| IBIS File LibisMaker.ibs
| LibisGen v2.0.1.0, 02/25/2008, Lattice Semiconductor Corporation
| Modified by LibisMaker v2.0.1.0, 02/25/2008, Lattice Semiconductor
| North Carolina State University, ERL, 2006
[IBIS ver]   3.2
[File name]   lptm21.ibs
[File Rev]   1.0
[Date]   May 27, 2015
[Source]   Lattice Semiconductor cs200fl Process
[Notes]   Device: LPTM21   Final
   Lattice Semiconductor has worked hard to ensure the
   models below are accurate and complete.  However, the
   data below was generated using simulation of the
   input/output model files for the silicon.  Therefore,
   the data below is for reference and initial design
   purposes only.
   Lattice Semiconductor grants permission to use this
   data for use in printed circuit design using this
   Lattice programmable logic device.  Other use of this
   code, including the selling or duplication of any
   portion is strictly prohibited.
|   NAMING CONVENTION
   The IBIS [Model] header is limited by the specification to a
   total of characters.  With such a set of characters available
   for naming models it becomes important to attempt to
   meaningfully encode the IO standards so they fit within the
   twenty character limit.  It would seem that twenty characters
   would provide room enough for describing IO's.  However, the
   PLD IO structure continues to grow more and more complex.  The
   complexity is making the twenty characters insuffiently
   descriptive.  In order to overcome this issue the naming
   convention described below is implemented to resolve the issue.
The twenty character space is managed as follows:
   bbbvvvsdddprugtcoixx
   b = standard
   v = voltage (x.xx V)
   s = slew code
   d = drive (xx.x ma)
   p = pullup code
   r = series resistance  or bank_vccio code
   u = terminate to vcc code
   g = terminate to gnd code
   t = terminate to vtt code
   c = common mode termination mode
   o = diff resistor code
   i = diff resistor current code
   x = reserved
   standard
   lvcmos   lvc
   lvcmosd   lvd
   lvcmosr   lvr
   lvds25e   lve
   lvttl   lvt
   lvttld   ltd
   pci   pci
   sstl_I   ss1
   sstl_II   ss2
   sstld_I   s1d
   sstld_II   s2d
   hstl_i   hs1
   hstl_ii   hs2
   hstld_i   h1d
   hstld_ii   h2d
   lvds25   lvs
   blvds25   blv
   blvds25e   blv
   mlvds25   mlv
   mlvds25e   mlv
   lvpecl33   lvp
   lvpecl33e   lvp
   rsds25   rsd
   rsds25e   rse
   mipi   mip
   mipi_lp   mip
   vref1   vr1
   vref2   vr2
   ref_res   rer
   slew
   na   a
   fast   f
   slow   s
   pullmode
   off   a
   pullup   b
   pulldown   c
   bushold   d
   clamp   e
   up_clamp   f
   down_clamp   g
   keeper_clamp   h
   impedance or Bank_vccio
   off   a
   25   b
   33   c
   50   d
   100   e
   3.3   f
   2.5   g
   1.8   h
   1.5   i
   1.2   j
   termVCC
   off   a
   50   b
   100   c
   120   d
   termGND
   off   a
   50   b
   100   c
   120   d
   termVTT
   off   a
   60   b
   75   c
   120   d
   150   e
   210   f
   VCMT
   off   a
   VCMT   b
   VTT   c
   DDR-2   d
   differential resistor
   off   a
   100   b
   diff drive
   NA   a
   2.0   b
   3.5   c
   1.25   f
   2.5   g
   Reserved   IO type
   in   input only
   ou   output
   io   I/O
   od   Open drain
   on   Inverting differential I/O
   (signal name only)
   op   Non-Inverting differential I/O
   (signal name only)
   Lattice Semiconductor Corporation
   5555 NE Moore Court
   Hillsboro, OR 97214
   U.S.A
   TEL: 1-800-Lattice (USA and Canada)
   408-826-6000 (other locations)
   web: http://www.latticesemi.com/
   email: techsupport@latticesemi.com
[Disclaimer] This IBIS source code is intended as a design reference
   which illustrates how the Lattice Semiconductor device operates.
   It is the user's responsibility to verify their design for
   consistency and functionality through the use of formal
   verification methods.  Lattice Semiconductor provides no warranty
   regarding the use or functionality of this data.
[Copyright]   Copyright 2007 by Lattice Semiconductor Corporation
|   Component LPTM21
[Component]   LPTM21
[Manufacturer]   Lattice Semiconductor Corp.
[Package]
|ftBGA237
| variable   typ   min   max
R_pkg   278.36m   251.54m   305.19m
L_pkg   6.04nH   3.27nH   8.79nH
C_pkg   0.509pF   0.44pF   0.704pF
[Pin] signal_name   model_name   R_pin   L_pin   C_pin
1   blv250axxxafaaaaaain   blv250axxxafaaaaaain
2   blv250axxxafaaaabain   blv250axxxafaaaabain
3   blv250axxxagaaaaaain   blv250axxxagaaaaaain
4   blv250axxxagaaaabain   blv250axxxagaaaabain
5   blv250axxxefaaaaaain   blv250axxxefaaaaaain
6   blv250axxxefaaaabain   blv250axxxefaaaabain
7   blv250axxxegaaaaaain   blv250axxxegaaaaaain
8   blv250axxxegaaaabain   blv250axxxegaaaabain
9   blv250f160aaaaaaaaio   blv250f160aaaaaaaaio
10   blv250f160aaaaaaaaop   blv250f160aaaaaaaaou
11   blv250f160aaaaaaaaon   blv250f160aaaaaaaaou
12   blv250f160eaaaaaaaio   blv250f160eaaaaaaaio
13   blv250f160eaaaaaaaop   blv250f160eaaaaaaaou
14   blv250f160eaaaaaaaon   blv250f160eaaaaaaaou
15   blv250s160aaaaaaaaio   blv250s160aaaaaaaaio
16   blv250s160aaaaaaaaop   blv250s160aaaaaaaaou
17   blv250s160aaaaaaaaon   blv250s160aaaaaaaaou
18   blv250s160eaaaaaaaio   blv250s160eaaaaaaaio
19   blv250s160eaaaaaaaop   blv250s160eaaaaaaaou
20   blv250s160eaaaaaaaon   blv250s160eaaaaaaaou
21   h1d180axxxafaaaaaain   h1d180axxxafaaaaaain
22   h1d180axxxafaaaabain   h1d180axxxafaaaabain
23   h1d180axxxagaaaaaain   h1d180axxxagaaaaaain
24   h1d180axxxagaaaabain   h1d180axxxagaaaabain
25   h1d180axxxahaaaaaain   h1d180axxxahaaaaaain
26   h1d180axxxahaaaabain   h1d180axxxahaaaabain
27   h1d180axxxefaaaaaain   h1d180axxxefaaaaaain
28   h1d180axxxefaaaabain   h1d180axxxefaaaabain
29   h1d180axxxegaaaaaain   h1d180axxxegaaaaaain
30   h1d180axxxegaaaabain   h1d180axxxegaaaabain
31   h1d180axxxehaaaaaain   h1d180axxxehaaaaaain
32   h1d180axxxehaaaabain   h1d180axxxehaaaabain
33   h1d180f080aaaaaaaaio   h1d180f080aaaaaaaaio
34   h1d180f080aaaaaaaaop   h1d180f080aaaaaaaaou
35   h1d180f080aaaaaaaaon   h1d180f080aaaaaaaaou
36   h1d180f080aaaaaabaio   h1d180f080aaaaaabaio
37   h1d180f080eaaaaaaaio   h1d180f080eaaaaaaaio
38   h1d180f080eaaaaaaaop   h1d180f080eaaaaaaaou
39   h1d180f080eaaaaaaaon   h1d180f080eaaaaaaaou
40   h1d180f080eaaaaabaio   h1d180f080eaaaaabaio
41   h1d180s080aaaaaaaaio   h1d180s080aaaaaaaaio
42   h1d180s080aaaaaaaaop   h1d180s080aaaaaaaaou
43   h1d180s080aaaaaaaaon   h1d180s080aaaaaaaaou
44   h1d180s080aaaaaabaio   h1d180s080aaaaaabaio
45   h1d180s080eaaaaaaaio   h1d180s080eaaaaaaaio
46   h1d180s080eaaaaaaaop   h1d180s080eaaaaaaaou
47   h1d180s080eaaaaaaaon   h1d180s080eaaaaaaaou
48   h1d180s080eaaaaabaio   h1d180s080eaaaaabaio
49   h2d180axxxafaaaaaain   h2d180axxxafaaaaaain
50   h2d180axxxafaaaabain   h2d180axxxafaaaabain
51   h2d180axxxagaaaaaain   h2d180axxxagaaaaaain
52   h2d180axxxagaaaabain   h2d180axxxagaaaabain
53   h2d180axxxahaaaaaain   h2d180axxxahaaaaaain
54   h2d180axxxahaaaabain   h2d180axxxahaaaabain
55   h2d180axxxefaaaaaain   h2d180axxxefaaaaaain
56   h2d180axxxefaaaabain   h2d180axxxefaaaabain
57   h2d180axxxegaaaaaain   h2d180axxxegaaaaaain
58   h2d180axxxegaaaabain   h2d180axxxegaaaabain
59   h2d180axxxehaaaaaain   h2d180axxxehaaaaaain
60   h2d180axxxehaaaabain   h2d180axxxehaaaabain
61   hs1180axxxafaaaaaain   hs1180axxxafaaaaaain
62   hs1180axxxagaaaaaain   hs1180axxxagaaaaaain
63   hs1180axxxahaaaaaain   hs1180axxxahaaaaaain
64   hs1180axxxefaaaaaain   hs1180axxxefaaaaaain
65   hs1180axxxegaaaaaain   hs1180axxxegaaaaaain
66   hs1180axxxehaaaaaain   hs1180axxxehaaaaaain
67   hs1180f080aaaaaaaaio   hs1180f080aaaaaaaaio
68   hs1180f080aaaaaaaaou   hs1180f080aaaaaaaaou
69   hs1180f080eaaaaaaaio   hs1180f080eaaaaaaaio
70   hs1180f080eaaaaaaaou   hs1180f080eaaaaaaaou
71   hs1180s080aaaaaaaaio   hs1180s080aaaaaaaaio
72   hs1180s080aaaaaaaaou   hs1180s080aaaaaaaaou
73   hs1180s080eaaaaaaaio   hs1180s080eaaaaaaaio
74   hs1180s080eaaaaaaaou   hs1180s080eaaaaaaaou
75   hs2180axxxafaaaaaain   hs2180axxxafaaaaaain
76   hs2180axxxagaaaaaain   hs2180axxxagaaaaaain
77   hs2180axxxahaaaaaain   hs2180axxxahaaaaaain
78   hs2180axxxefaaaaaain   hs2180axxxefaaaaaain
79   hs2180axxxegaaaaaain   hs2180axxxegaaaaaain
80   hs2180axxxehaaaaaain   hs2180axxxehaaaaaain
81   ltd330axxxafaaaaaain   ltd330axxxafaaaaaain
82   ltd330axxxefaaaaaain   ltd330axxxefaaaaaain
83   ltd330f040aaaaaaaaio   ltd330f040aaaaaaaaio
84   ltd330f040aaaaaaaaop   ltd330f040aaaaaaaaou
85   ltd330f040aaaaaaaaon   ltd330f040aaaaaaaaou
86   ltd330f040eaaaaaaaio   ltd330f040eaaaaaaaio
87   ltd330f040eaaaaaaaop   ltd330f040eaaaaaaaou
88   ltd330f040eaaaaaaaon   ltd330f040eaaaaaaaou
89   ltd330f080aaaaaaaaio   ltd330f080aaaaaaaaio
90   ltd330f080aaaaaaaaop   ltd330f080aaaaaaaaou
91   ltd330f080aaaaaaaaon   ltd330f080aaaaaaaaou
92   ltd330f080eaaaaaaaio   ltd330f080eaaaaaaaio
93   ltd330f080eaaaaaaaop   ltd330f080eaaaaaaaou
94   ltd330f080eaaaaaaaon   ltd330f080eaaaaaaaou
95   ltd330f120aaaaaaaaio   ltd330f120aaaaaaaaio
96   ltd330f120aaaaaaaaop   ltd330f120aaaaaaaaou
97   ltd330f120aaaaaaaaon   ltd330f120aaaaaaaaou
98   ltd330f120eaaaaaaaio   ltd330f120eaaaaaaaio
99   ltd330f120eaaaaaaaop   ltd330f120eaaaaaaaou
100  ltd330f120eaaaaaaaon   ltd330f120eaaaaaaaou
101  ltd330f160aaaaaaaaio   ltd330f160aaaaaaaaio
102  ltd330f160aaaaaaaaop   ltd330f160aaaaaaaaou
103  ltd330f160aaaaaaaaon   ltd330f160aaaaaaaaou
104  ltd330f160eaaaaaaaio   ltd330f160eaaaaaaaio
105  ltd330f160eaaaaaaaop   ltd330f160eaaaaaaaou
106  ltd330f160eaaaaaaaon   ltd330f160eaaaaaaaou
107  ltd330f240aaaaaaaaio   ltd330f240aaaaaaaaio
108  ltd330f240aaaaaaaaop   ltd330f240aaaaaaaaou
109  ltd330f240aaaaaaaaon   ltd330f240aaaaaaaaou
110  ltd330f240eaaaaaaaio   ltd330f240eaaaaaaaio
111  ltd330f240eaaaaaaaop   ltd330f240eaaaaaaaou
112  ltd330f240eaaaaaaaon   ltd330f240eaaaaaaaou
113  ltd330s040aaaaaaaaio   ltd330s040aaaaaaaaio
114  ltd330s040aaaaaaaaop   ltd330s040aaaaaaaaou
115  ltd330s040aaaaaaaaon   ltd330s040aaaaaaaaou
116  ltd330s040eaaaaaaaio   ltd330s040eaaaaaaaio
117  ltd330s040eaaaaaaaop   ltd330s040eaaaaaaaou
118  ltd330s040eaaaaaaaon   ltd330s040eaaaaaaaou
119  ltd330s080aaaaaaaaio   ltd330s080aaaaaaaaio
120  ltd330s080aaaaaaaaop   ltd330s080aaaaaaaaou
121  ltd330s080aaaaaaaaon   ltd330s080aaaaaaaaou
122  ltd330s080eaaaaaaaio   ltd330s080eaaaaaaaio
123  ltd330s080eaaaaaaaop   ltd330s080eaaaaaaaou
124  ltd330s080eaaaaaaaon   ltd330s080eaaaaaaaou
125  ltd330s120aaaaaaaaio   ltd330s120aaaaaaaaio
126  ltd330s120aaaaaaaaop   ltd330s120aaaaaaaaou
127  ltd330s120aaaaaaaaon   ltd330s120aaaaaaaaou
128  ltd330s120eaaaaaaaio   ltd330s120eaaaaaaaio
129  ltd330s120eaaaaaaaop   ltd330s120eaaaaaaaou
130  ltd330s120eaaaaaaaon   ltd330s120eaaaaaaaou
131  ltd330s160aaaaaaaaio   ltd330s160aaaaaaaaio
132  ltd330s160aaaaaaaaop   ltd330s160aaaaaaaaou
133  ltd330s160aaaaaaaaon   ltd330s160aaaaaaaaou
134  ltd330s160eaaaaaaaio   ltd330s160eaaaaaaaio
135  ltd330s160eaaaaaaaop   ltd330s160eaaaaaaaou
136  ltd330s160eaaaaaaaon   ltd330s160eaaaaaaaou
137  ltd330s240aaaaaaaaio   ltd330s240aaaaaaaaio
138  ltd330s240aaaaaaaaop   ltd330s240aaaaaaaaou
139  ltd330s240aaaaaaaaon   ltd330s240aaaaaaaaou
140  ltd330s240eaaaaaaaio   ltd330s240eaaaaaaaio
141  ltd330s240eaaaaaaaop   ltd330s240eaaaaaaaou
142  ltd330s240eaaaaaaaon   ltd330s240eaaaaaaaou
143  lvc120axxxafaaaaaain   lvc120axxxafaaaaaain
144  lvc120axxxagaaaaaain   lvc120axxxagaaaaaain
145  lvc120axxxahaaaaaain   lvc120axxxahaaaaaain
146  lvc120axxxaiaaaaaain   lvc120axxxaiaaaaaain
147  lvc120axxxbjaaaaaain   lvc120axxxbjaaaaaain
148  lvc120axxxcfaaaaaain   lvc120axxxcfaaaaaain
149  lvc120axxxcgaaaaaain   lvc120axxxcgaaaaaain
150  lvc120axxxchaaaaaain   lvc120axxxchaaaaaain
151  lvc120axxxciaaaaaain   lvc120axxxciaaaaaain
152  lvc120axxxdjaaaaaain   lvc120axxxdjaaaaaain
153  lvc120axxxefaaaaaain   lvc120axxxefaaaaaain
154  lvc120axxxegaaaaaain   lvc120axxxegaaaaaain
155  lvc120axxxehaaaaaain   lvc120axxxehaaaaaain
156  lvc120axxxeiaaaaaain   lvc120axxxeiaaaaaain
157  lvc120axxxejaaaaaain   lvc120axxxejaaaaaain
158  lvc120axxxfjaaaaaain   lvc120axxxfjaaaaaain
159  lvc120axxxgfaaaaaain   lvc120axxxgfaaaaaain
160  lvc120axxxggaaaaaain   lvc120axxxggaaaaaain
161  lvc120axxxghaaaaaain   lvc120axxxghaaaaaain
162  lvc120axxxgiaaaaaain   lvc120axxxgiaaaaaain
163  lvc120axxxgjaaaaaain   lvc120axxxgjaaaaaain
164  lvc120axxxhjaaaaaain   lvc120axxxhjaaaaaain
165  lvc120f020aaaaaaaaio   lvc120f020aaaaaaaaio
166  lvc120f020aaaaaaaaou   lvc120f020aaaaaaaaou
167  lvc120f020baaaaaaaio   lvc120f020baaaaaaaio
168  lvc120f020baaaaaaaou   lvc120f020baaaaaaaou
169  lvc120f020caaaaaaaio   lvc120f020caaaaaaaio
170  lvc120f020caaaaaaaou   lvc120f020caaaaaaaou
171  lvc120f020daaaaaaaio   lvc120f020daaaaaaaio
172  lvc120f020daaaaaaaou   lvc120f020daaaaaaaou
173  lvc120f020eaaaaaaaio   lvc120f020eaaaaaaaio
174  lvc120f020eaaaaaaaou   lvc120f020eaaaaaaaou
175  lvc120f020faaaaaaaio   lvc120f020faaaaaaaio
176  lvc120f020faaaaaaaou   lvc120f020faaaaaaaou
177  lvc120f020gaaaaaaaio   lvc120f020gaaaaaaaio
178  lvc120f020gaaaaaaaou   lvc120f020gaaaaaaaou
179  lvc120f020haaaaaaaio   lvc120f020haaaaaaaio
180  lvc120f020haaaaaaaou   lvc120f020haaaaaaaou
181  lvc120f040afaaaaaaod   lvc120f040afaaaaaaod
182  lvc120f040agaaaaaaod   lvc120f040agaaaaaaod
183  lvc120f040ahaaaaaaod   lvc120f040ahaaaaaaod
184  lvc120f040aiaaaaaaod   lvc120f040aiaaaaaaod
185  lvc120f040ajaaaaaaod   lvc120f040ajaaaaaaod
186  lvc120f060aaaaaaaaio   lvc120f060aaaaaaaaio
187  lvc120f060aaaaaaaaou   lvc120f060aaaaaaaaou
188  lvc120f060baaaaaaaio   lvc120f060baaaaaaaio
189  lvc120f060baaaaaaaou   lvc120f060baaaaaaaou
190  lvc120f060caaaaaaaio   lvc120f060caaaaaaaio
191  lvc120f060caaaaaaaou   lvc120f060caaaaaaaou
192  lvc120f060daaaaaaaio   lvc120f060daaaaaaaio
193  lvc120f060daaaaaaaou   lvc120f060daaaaaaaou
194  lvc120f060eaaaaaaaio   lvc120f060eaaaaaaaio
195  lvc120f060eaaaaaaaou   lvc120f060eaaaaaaaou
196  lvc120f060faaaaaaaio   lvc120f060faaaaaaaio
197  lvc120f060faaaaaaaou   lvc120f060faaaaaaaou
198  lvc120f060gaaaaaaaio   lvc120f060gaaaaaaaio
199  lvc120f060gaaaaaaaou   lvc120f060gaaaaaaaou
200  lvc120f060haaaaaaaio   lvc120f060haaaaaaaio
201  lvc120f060haaaaaaaou   lvc120f060haaaaaaaou
202  lvc120f080afaaaaaaod   lvc120f080afaaaaaaod
203  lvc120f080agaaaaaaod   lvc120f080agaaaaaaod
204  lvc120f080ahaaaaaaod   lvc120f080ahaaaaaaod
205  lvc120f080aiaaaaaaod   lvc120f080aiaaaaaaod
206  lvc120f080ajaaaaaaod   lvc120f080ajaaaaaaod
207  lvc120f120afaaaaaaod   lvc120f120afaaaaaaod
208  lvc120f120agaaaaaaod   lvc120f120agaaaaaaod
209  lvc120f120ahaaaaaaod   lvc120f120ahaaaaaaod
210  lvc120f160afaaaaaaod   lvc120f160afaaaaaaod
211  lvc120f160agaaaaaaod   lvc120f160agaaaaaaod
212  lvc120f240afaaaaaaod   lvc120f240afaaaaaaod
213  lvc120s020aaaaaaaaio   lvc120s020aaaaaaaaio
214  lvc120s020aaaaaaaaou   lvc120s020aaaaaaaaou
215  lvc120s020baaaaaaaio   lvc120s020baaaaaaaio
216  lvc120s020baaaaaaaou   lvc120s020baaaaaaaou
217  lvc120s020caaaaaaaio   lvc120s020caaaaaaaio
218  lvc120s020caaaaaaaou   lvc120s020caaaaaaaou
219  lvc120s020daaaaaaaio   lvc120s020daaaaaaaio
220  lvc120s020daaaaaaaou   lvc120s020daaaaaaaou
221  lvc120s020eaaaaaaaio   lvc120s020eaaaaaaaio
222  lvc120s020eaaaaaaaou   lvc120s020eaaaaaaaou
223  lvc120s020faaaaaaaio   lvc120s020faaaaaaaio
224  lvc120s020faaaaaaaou   lvc120s020faaaaaaaou
225  lvc120s020gaaaaaaaio   lvc120s020gaaaaaaaio
226  lvc120s020gaaaaaaaou   lvc120s020gaaaaaaaou
227  lvc120s020haaaaaaaio   lvc120s020haaaaaaaio
228  lvc120s020haaaaaaaou   lvc120s020haaaaaaaou
229  lvc120s040afaaaaaaod   lvc120s040afaaaaaaod
230  lvc120s040agaaaaaaod   lvc120s040agaaaaaaod
231  lvc120s040ahaaaaaaod   lvc120s040ahaaaaaaod
232  lvc120s040aiaaaaaaod   lvc120s040aiaaaaaaod
233  lvc120s040ajaaaaaaod   lvc120s040ajaaaaaaod
234  lvc120s060aaaaaaaaio   lvc120s060aaaaaaaaio
235  lvc120s060aaaaaaaaou   lvc120s060aaaaaaaaou
236  lvc120s060baaaaaaaio   lvc120s060baaaaaaaio
237  lvc120s060baaaaaaaou   lvc120s060baaaaaaaou
238  lvc120s060caaaaaaaio   lvc120s060caaaaaaaio
239  lvc120s060caaaaaaaou   lvc120s060caaaaaaaou
240  lvc120s060daaaaaaaio   lvc120s060daaaaaaaio
241  lvc120s060daaaaaaaou   lvc120s060daaaaaaaou
242  lvc120s060eaaaaaaaio   lvc120s060eaaaaaaaio
243  lvc120s060eaaaaaaaou   lvc120s060eaaaaaaaou
244  lvc120s060faaaaaaaio   lvc120s060faaaaaaaio
245  lvc120s060faaaaaaaou   lvc120s060faaaaaaaou
246  lvc120s060gaaaaaaaio   lvc120s060gaaaaaaaio
247  lvc120s060gaaaaaaaou   lvc120s060gaaaaaaaou
248  lvc120s060haaaaaaaio   lvc120s060haaaaaaaio
249  lvc120s060haaaaaaaou   lvc120s060haaaaaaaou
250  lvc120s080afaaaaaaod   lvc120s080afaaaaaaod
251  lvc120s080agaaaaaaod   lvc120s080agaaaaaaod
252  lvc120s080ahaaaaaaod   lvc120s080ahaaaaaaod
253  lvc120s080aiaaaaaaod   lvc120s080aiaaaaaaod
254  lvc120s080ajaaaaaaod   lvc120s080ajaaaaaaod
255  lvc120s120afaaaaaaod   lvc120s120afaaaaaaod
256  lvc120s120agaaaaaaod   lvc120s120agaaaaaaod
257  lvc120s120ahaaaaaaod   lvc120s120ahaaaaaaod
258  lvc120s160afaaaaaaod   lvc120s160afaaaaaaod
259  lvc120s160agaaaaaaod   lvc120s160agaaaaaaod
260  lvc120s240afaaaaaaod   lvc120s240afaaaaaaod
261  lvc150axxxafaaaaaain   lvc150axxxafaaaaaain
262  lvc150axxxagaaaaaain   lvc150axxxagaaaaaain
263  lvc150axxxahaaaaaain   lvc150axxxahaaaaaain
264  lvc150axxxaiaaaaaain   lvc150axxxaiaaaaaain
265  lvc150axxxajaaaaaain   lvc150axxxajaaaaaain
266  lvc150axxxbiaaaaaain   lvc150axxxbiaaaaaain
267  lvc150axxxcfaaaaaain   lvc150axxxcfaaaaaain
268  lvc150axxxcgaaaaaain   lvc150axxxcgaaaaaain
269  lvc150axxxchaaaaaain   lvc150axxxchaaaaaain
270  lvc150axxxciaaaaaain   lvc150axxxciaaaaaain
271  lvc150axxxcjaaaaaain   lvc150axxxcjaaaaaain
272  lvc150axxxdiaaaaaain   lvc150axxxdiaaaaaain
273  lvc150axxxefaaaaaain   lvc150axxxefaaaaaain
274  lvc150axxxegaaaaaain   lvc150axxxegaaaaaain
275  lvc150axxxehaaaaaain   lvc150axxxehaaaaaain
276  lvc150axxxeiaaaaaain   lvc150axxxeiaaaaaain
277  lvc150axxxfiaaaaaain   lvc150axxxfiaaaaaain
278  lvc150axxxgfaaaaaain   lvc150axxxgfaaaaaain
279  lvc150axxxggaaaaaain   lvc150axxxggaaaaaain
280  lvc150axxxghaaaaaain   lvc150axxxghaaaaaain
281  lvc150axxxgiaaaaaain   lvc150axxxgiaaaaaain
282  lvc150axxxhiaaaaaain   lvc150axxxhiaaaaaain
283  lvc150f040aaaaaaaaio   lvc150f040aaaaaaaaio
284  lvc150f040aaaaaaaaou   lvc150f040aaaaaaaaou
285  lvc150f040afaaaaaaod   lvc150f040afaaaaaaod
286  lvc150f040agaaaaaaod   lvc150f040agaaaaaaod
287  lvc150f040ahaaaaaaod   lvc150f040ahaaaaaaod
288  lvc150f040aiaaaaaaod   lvc150f040aiaaaaaaod
289  lvc150f040ajaaaaaaod   lvc150f040ajaaaaaaod
290  lvc150f040baaaaaaaio   lvc150f040baaaaaaaio
291  lvc150f040baaaaaaaou   lvc150f040baaaaaaaou
292  lvc150f040caaaaaaaio   lvc150f040caaaaaaaio
293  lvc150f040caaaaaaaou   lvc150f040caaaaaaaou
294  lvc150f040daaaaaaaio   lvc150f040daaaaaaaio
295  lvc150f040daaaaaaaou   lvc150f040daaaaaaaou
296  lvc150f040eaaaaaaaio   lvc150f040eaaaaaaaio
297  lvc150f040eaaaaaaaou   lvc150f040eaaaaaaaou
298  lvc150f040faaaaaaaio   lvc150f040faaaaaaaio
299  lvc150f040faaaaaaaou   lvc150f040faaaaaaaou
300  lvc150f040gaaaaaaaio   lvc150f040gaaaaaaaio
301  lvc150f040gaaaaaaaou   lvc150f040gaaaaaaaou
302  lvc150f040haaaaaaaio   lvc150f040haaaaaaaio
303  lvc150f040haaaaaaaou   lvc150f040haaaaaaaou
304  lvc150f080aaaaaaaaio   lvc150f080aaaaaaaaio
305  lvc150f080aaaaaaaaou   lvc150f080aaaaaaaaou
306  lvc150f080afaaaaaaod   lvc150f080afaaaaaaod
307  lvc150f080agaaaaaaod   lvc150f080agaaaaaaod
308  lvc150f080ahaaaaaaod   lvc150f080ahaaaaaaod
309  lvc150f080aiaaaaaaod   lvc150f080aiaaaaaaod
310  lvc150f080ajaaaaaaod   lvc150f080ajaaaaaaod
311  lvc150f080baaaaaaaio   lvc150f080baaaaaaaio
312  lvc150f080baaaaaaaou   lvc150f080baaaaaaaou
313  lvc150f080caaaaaaaio   lvc150f080caaaaaaaio
314  lvc150f080caaaaaaaou   lvc150f080caaaaaaaou
315  lvc150f080daaaaaaaio   lvc150f080daaaaaaaio
316  lvc150f080daaaaaaaou   lvc150f080daaaaaaaou
317  lvc150f080eaaaaaaaio   lvc150f080eaaaaaaaio
318  lvc150f080eaaaaaaaou   lvc150f080eaaaaaaaou
319  lvc150f080faaaaaaaio   lvc150f080faaaaaaaio
320  lvc150f080faaaaaaaou   lvc150f080faaaaaaaou
321  lvc150f080gaaaaaaaio   lvc150f080gaaaaaaaio
322  lvc150f080gaaaaaaaou   lvc150f080gaaaaaaaou
323  lvc150f080haaaaaaaio   lvc150f080haaaaaaaio
324  lvc150f080haaaaaaaou   lvc150f080haaaaaaaou
325  lvc150f120afaaaaaaod   lvc150f120afaaaaaaod
326  lvc150f120agaaaaaaod   lvc150f120agaaaaaaod
327  lvc150f120ahaaaaaaod   lvc150f120ahaaaaaaod
328  lvc150f160afaaaaaaod   lvc150f160afaaaaaaod
329  lvc150f160agaaaaaaod   lvc150f160agaaaaaaod
330  lvc150f240afaaaaaaod   lvc150f240afaaaaaaod
331  lvc150s040aaaaaaaaio   lvc150s040aaaaaaaaio
332  lvc150s040aaaaaaaaou   lvc150s040aaaaaaaaou
333  lvc150s040afaaaaaaod   lvc150s040afaaaaaaod
334  lvc150s040agaaaaaaod   lvc150s040agaaaaaaod
335  lvc150s040ahaaaaaaod   lvc150s040ahaaaaaaod
336  lvc150s040aiaaaaaaod   lvc150s040aiaaaaaaod
337  lvc150s040ajaaaaaaod   lvc150s040ajaaaaaaod
338  lvc150s040baaaaaaaio   lvc150s040baaaaaaaio
339  lvc150s040baaaaaaaou   lvc150s040baaaaaaaou
340  lvc150s040caaaaaaaio   lvc150s040caaaaaaaio
341  lvc150s040caaaaaaaou   lvc150s040caaaaaaaou
342  lvc150s040daaaaaaaio   lvc150s040daaaaaaaio
343  lvc150s040daaaaaaaou   lvc150s040daaaaaaaou
344  lvc150s040eaaaaaaaio   lvc150s040eaaaaaaaio
345  lvc150s040eaaaaaaaou   lvc150s040eaaaaaaaou
346  lvc150s040faaaaaaaio   lvc150s040faaaaaaaio
347  lvc150s040faaaaaaaou   lvc150s040faaaaaaaou
348  lvc150s040gaaaaaaaio   lvc150s040gaaaaaaaio
349  lvc150s040gaaaaaaaou   lvc150s040gaaaaaaaou
350  lvc150s040haaaaaaaio   lvc150s040haaaaaaaio
351  lvc150s040haaaaaaaou   lvc150s040haaaaaaaou
352  lvc150s080aaaaaaaaio   lvc150s080aaaaaaaaio
353  lvc150s080aaaaaaaaou   lvc150s080aaaaaaaaou
354  lvc150s080afaaaaaaod   lvc150s080afaaaaaaod
355  lvc150s080agaaaaaaod   lvc150s080agaaaaaaod
356  lvc150s080ahaaaaaaod   lvc150s080ahaaaaaaod
357  lvc150s080aiaaaaaaod   lvc150s080aiaaaaaaod
358  lvc150s080ajaaaaaaod   lvc150s080ajaaaaaaod
359  lvc150s080baaaaaaaio   lvc150s080baaaaaaaio
360  lvc150s080baaaaaaaou   lvc150s080baaaaaaaou
361  lvc150s080caaaaaaaio   lvc150s080caaaaaaaio
362  lvc150s080caaaaaaaou   lvc150s080caaaaaaaou
363  lvc150s080daaaaaaaio   lvc150s080daaaaaaaio
364  lvc150s080daaaaaaaou   lvc150s080daaaaaaaou
365  lvc150s080eaaaaaaaio   lvc150s080eaaaaaaaio
366  lvc150s080eaaaaaaaou   lvc150s080eaaaaaaaou
367  lvc150s080faaaaaaaio   lvc150s080faaaaaaaio
368  lvc150s080faaaaaaaou   lvc150s080faaaaaaaou
369  lvc150s080gaaaaaaaio   lvc150s080gaaaaaaaio
370  lvc150s080gaaaaaaaou   lvc150s080gaaaaaaaou
371  lvc150s080haaaaaaaio   lvc150s080haaaaaaaio
372  lvc150s080haaaaaaaou   lvc150s080haaaaaaaou
373  lvc150s120afaaaaaaod   lvc150s120afaaaaaaod
374  lvc150s120agaaaaaaod   lvc150s120agaaaaaaod
375  lvc150s120ahaaaaaaod   lvc150s120ahaaaaaaod
376  lvc150s160afaaaaaaod   lvc150s160afaaaaaaod
377  lvc150s160agaaaaaaod   lvc150s160agaaaaaaod
378  lvc150s240afaaaaaaod   lvc150s240afaaaaaaod
379  lvc180axxxafaaaaaain   lvc180axxxafaaaaaain
380  lvc180axxxagaaaaaain   lvc180axxxagaaaaaain
381  lvc180axxxahaaaaaain   lvc180axxxahaaaaaain
382  lvc180axxxaiaaaaaain   lvc180axxxaiaaaaaain
383  lvc180axxxbhaaaaaain   lvc180axxxbhaaaaaain
384  lvc180axxxcfaaaaaain   lvc180axxxcfaaaaaain
385  lvc180axxxcgaaaaaain   lvc180axxxcgaaaaaain
386  lvc180axxxchaaaaaain   lvc180axxxchaaaaaain
387  lvc180axxxciaaaaaain   lvc180axxxciaaaaaain
388  lvc180axxxdhaaaaaain   lvc180axxxdhaaaaaain
389  lvc180axxxefaaaaaain   lvc180axxxefaaaaaain
390  lvc180axxxegaaaaaain   lvc180axxxegaaaaaain
391  lvc180axxxehaaaaaain   lvc180axxxehaaaaaain
392  lvc180axxxfhaaaaaain   lvc180axxxfhaaaaaain
393  lvc180axxxgfaaaaaain   lvc180axxxgfaaaaaain
394  lvc180axxxggaaaaaain   lvc180axxxggaaaaaain
395  lvc180axxxghaaaaaain   lvc180axxxghaaaaaain
396  lvc180axxxhhaaaaaain   lvc180axxxhhaaaaaain
397  lvc180f040aaaaaaaaio   lvc180f040aaaaaaaaio
398  lvc180f040aaaaaaaaou   lvc180f040aaaaaaaaou
399  lvc180f040afaaaaaaod   lvc180f040afaaaaaaod
400  lvc180f040agaaaaaaod   lvc180f040agaaaaaaod
401  lvc180f040ahaaaaaaod   lvc180f040ahaaaaaaod
402  lvc180f040aiaaaaaaod   lvc180f040aiaaaaaaod
403  lvc180f040ajaaaaaaod   lvc180f040ajaaaaaaod
404  lvc180f040baaaaaaaio   lvc180f040baaaaaaaio
405  lvc180f040baaaaaaaou   lvc180f040baaaaaaaou
406  lvc180f040caaaaaaaio   lvc180f040caaaaaaaio
407  lvc180f040caaaaaaaou   lvc180f040caaaaaaaou
408  lvc180f040daaaaaaaio   lvc180f040daaaaaaaio
409  lvc180f040daaaaaaaou   lvc180f040daaaaaaaou
410  lvc180f040eaaaaaaaio   lvc180f040eaaaaaaaio
411  lvc180f040eaaaaaaaou   lvc180f040eaaaaaaaou
412  lvc180f040faaaaaaaio   lvc180f040faaaaaaaio
413  lvc180f040faaaaaaaou   lvc180f040faaaaaaaou
414  lvc180f040gaaaaaaaio   lvc180f040gaaaaaaaio
415  lvc180f040gaaaaaaaou   lvc180f040gaaaaaaaou
416  lvc180f040haaaaaaaio   lvc180f040haaaaaaaio
417  lvc180f040haaaaaaaou   lvc180f040haaaaaaaou
418  lvc180f080aaaaaaaaio   lvc180f080aaaaaaaaio
419  lvc180f080aaaaaaaaou   lvc180f080aaaaaaaaou
420  lvc180f080afaaaaaaod   lvc180f080afaaaaaaod
421  lvc180f080agaaaaaaod   lvc180f080agaaaaaaod
422  lvc180f080ahaaaaaaod   lvc180f080ahaaaaaaod
423  lvc180f080aiaaaaaaod   lvc180f080aiaaaaaaod
424  lvc180f080ajaaaaaaod   lvc180f080ajaaaaaaod
425  lvc180f080baaaaaaaio   lvc180f080baaaaaaaio
426  lvc180f080baaaaaaaou   lvc180f080baaaaaaaou
427  lvc180f080caaaaaaaio   lvc180f080caaaaaaaio
428  lvc180f080caaaaaaaou   lvc180f080caaaaaaaou
429  lvc180f080daaaaaaaio   lvc180f080daaaaaaaio
430  lvc180f080daaaaaaaou   lvc180f080daaaaaaaou
431  lvc180f080eaaaaaaaio   lvc180f080eaaaaaaaio
432  lvc180f080eaaaaaaaou   lvc180f080eaaaaaaaou
433  lvc180f080faaaaaaaio   lvc180f080faaaaaaaio
434  lvc180f080faaaaaaaou   lvc180f080faaaaaaaou
435  lvc180f080gaaaaaaaio   lvc180f080gaaaaaaaio
436  lvc180f080gaaaaaaaou   lvc180f080gaaaaaaaou
437  lvc180f080haaaaaaaio   lvc180f080haaaaaaaio
438  lvc180f080haaaaaaaou   lvc180f080haaaaaaaou
439  lvc180f120aaaaaaaaio   lvc180f120aaaaaaaaio
440  lvc180f120aaaaaaaaou   lvc180f120aaaaaaaaou
441  lvc180f120afaaaaaaod   lvc180f120afaaaaaaod
442  lvc180f120agaaaaaaod   lvc180f120agaaaaaaod
443  lvc180f120ahaaaaaaod   lvc180f120ahaaaaaaod
444  lvc180f120baaaaaaaio   lvc180f120baaaaaaaio
445  lvc180f120baaaaaaaou   lvc180f120baaaaaaaou
446  lvc180f120caaaaaaaio   lvc180f120caaaaaaaio
447  lvc180f120caaaaaaaou   lvc180f120caaaaaaaou
448  lvc180f120daaaaaaaio   lvc180f120daaaaaaaio
449  lvc180f120daaaaaaaou   lvc180f120daaaaaaaou
450  lvc180f120eaaaaaaaio   lvc180f120eaaaaaaaio
451  lvc180f120eaaaaaaaou   lvc180f120eaaaaaaaou
452  lvc180f120faaaaaaaio   lvc180f120faaaaaaaio
453  lvc180f120faaaaaaaou   lvc180f120faaaaaaaou
454  lvc180f120gaaaaaaaio   lvc180f120gaaaaaaaio
455  lvc180f120gaaaaaaaou   lvc180f120gaaaaaaaou
456  lvc180f120haaaaaaaio   lvc180f120haaaaaaaio
457  lvc180f120haaaaaaaou   lvc180f120haaaaaaaou
458  lvc180f160afaaaaaaod   lvc180f160afaaaaaaod
459  lvc180f160agaaaaaaod   lvc180f160agaaaaaaod
460  lvc180f240afaaaaaaod   lvc180f240afaaaaaaod
461  lvc180s040aaaaaaaaio   lvc180s040aaaaaaaaio
462  lvc180s040aaaaaaaaou   lvc180s040aaaaaaaaou
463  lvc180s040afaaaaaaod   lvc180s040afaaaaaaod
464  lvc180s040agaaaaaaod   lvc180s040agaaaaaaod
465  lvc180s040ahaaaaaaod   lvc180s040ahaaaaaaod
466  lvc180s040aiaaaaaaod   lvc180s040aiaaaaaaod
467  lvc180s040ajaaaaaaod   lvc180s040ajaaaaaaod
468  lvc180s040baaaaaaaio   lvc180s040baaaaaaaio
469  lvc180s040baaaaaaaou   lvc180s040baaaaaaaou
470  lvc180s040caaaaaaaio   lvc180s040caaaaaaaio
471  lvc180s040caaaaaaaou   lvc180s040caaaaaaaou
472  lvc180s040daaaaaaaio   lvc180s040daaaaaaaio
473  lvc180s040daaaaaaaou   lvc180s040daaaaaaaou
474  lvc180s040eaaaaaaaio   lvc180s040eaaaaaaaio
475  lvc180s040eaaaaaaaou   lvc180s040eaaaaaaaou
476  lvc180s040faaaaaaaio   lvc180s040faaaaaaaio
477  lvc180s040faaaaaaaou   lvc180s040faaaaaaaou
478  lvc180s040gaaaaaaaio   lvc180s040gaaaaaaaio
479  lvc180s040gaaaaaaaou   lvc180s040gaaaaaaaou
480  lvc180s040haaaaaaaio   lvc180s040haaaaaaaio
481  lvc180s040haaaaaaaou   lvc180s040haaaaaaaou
482  lvc180s080aaaaaaaaio   lvc180s080aaaaaaaaio
483  lvc180s080aaaaaaaaou   lvc180s080aaaaaaaaou
484  lvc180s080afaaaaaaod   lvc180s080afaaaaaaod
485  lvc180s080agaaaaaaod   lvc180s080agaaaaaaod
486  lvc180s080ahaaaaaaod   lvc180s080ahaaaaaaod
487  lvc180s080aiaaaaaaod   lvc180s080aiaaaaaaod
488  lvc180s080ajaaaaaaod   lvc180s080ajaaaaaaod
489  lvc180s080baaaaaaaio   lvc180s080baaaaaaaio
490  lvc180s080baaaaaaaou   lvc180s080baaaaaaaou
491  lvc180s080caaaaaaaio   lvc180s080caaaaaaaio
492  lvc180s080caaaaaaaou   lvc180s080caaaaaaaou
493  lvc180s080daaaaaaaio   lvc180s080daaaaaaaio
494  lvc180s080daaaaaaaou   lvc180s080daaaaaaaou
495  lvc180s080eaaaaaaaio   lvc180s080eaaaaaaaio
496  lvc180s080eaaaaaaaou   lvc180s080eaaaaaaaou
497  lvc180s080faaaaaaaio   lvc180s080faaaaaaaio
498  lvc180s080faaaaaaaou   lvc180s080faaaaaaaou
499  lvc180s080gaaaaaaaio   lvc180s080gaaaaaaaio
500  lvc180s080gaaaaaaaou   lvc180s080gaaaaaaaou
501  lvc180s080haaaaaaaio   lvc180s080haaaaaaaio
502  lvc180s080haaaaaaaou   lvc180s080haaaaaaaou
503  lvc180s120aaaaaaaaio   lvc180s120aaaaaaaaio
504  lvc180s120aaaaaaaaou   lvc180s120aaaaaaaaou
505  lvc180s120afaaaaaaod   lvc180s120afaaaaaaod
506  lvc180s120agaaaaaaod   lvc180s120agaaaaaaod
507  lvc180s120ahaaaaaaod   lvc180s120ahaaaaaaod
508  lvc180s120baaaaaaaio   lvc180s120baaaaaaaio
509  lvc180s120baaaaaaaou   lvc180s120baaaaaaaou
510  lvc180s120caaaaaaaio   lvc180s120caaaaaaaio
511  lvc180s120caaaaaaaou   lvc180s120caaaaaaaou
512  lvc180s120daaaaaaaio   lvc180s120daaaaaaaio
513  lvc180s120daaaaaaaou   lvc180s120daaaaaaaou
514  lvc180s120eaaaaaaaio   lvc180s120eaaaaaaaio
515  lvc180s120eaaaaaaaou   lvc180s120eaaaaaaaou
516  lvc180s120faaaaaaaio   lvc180s120faaaaaaaio
517  lvc180s120faaaaaaaou   lvc180s120faaaaaaaou
518  lvc180s120gaaaaaaaio   lvc180s120gaaaaaaaio
519  lvc180s120gaaaaaaaou   lvc180s120gaaaaaaaou
520  lvc180s120haaaaaaaio   lvc180s120haaaaaaaio
521  lvc180s120haaaaaaaou   lvc180s120haaaaaaaou
522  lvc180s160afaaaaaaod   lvc180s160afaaaaaaod
523  lvc180s160agaaaaaaod   lvc180s160agaaaaaaod
524  lvc180s240afaaaaaaod   lvc180s240afaaaaaaod
525  lvc250axxxafaaaaaain   lvc250axxxafaaaaaain
526  lvc250axxxagaaaaaain   lvc250axxxagaaaaaain
527  lvc250axxxahaaaaaain   lvc250axxxahaaaaaain
528  lvc250axxxaiaaaaaain   lvc250axxxaiaaaaaain
529  lvc250axxxbgaaaaaain   lvc250axxxbgaaaaaain
530  lvc250axxxcfaaaaaain   lvc250axxxcfaaaaaain
531  lvc250axxxcgaaaaaain   lvc250axxxcgaaaaaain
532  lvc250axxxchaaaaaain   lvc250axxxchaaaaaain
533  lvc250axxxciaaaaaain   lvc250axxxciaaaaaain
534  lvc250axxxdgaaaaaain   lvc250axxxdgaaaaaain
535  lvc250axxxefaaaaaain   lvc250axxxefaaaaaain
536  lvc250axxxegaaaaaain   lvc250axxxegaaaaaain
537  lvc250axxxfgaaaaaain   lvc250axxxfgaaaaaain
538  lvc250axxxgfaaaaaain   lvc250axxxgfaaaaaain
539  lvc250axxxggaaaaaain   lvc250axxxggaaaaaain
540  lvc250axxxhgaaaaaain   lvc250axxxhgaaaaaain
541  lvc250f040aaaaaaaaio   lvc250f040aaaaaaaaio
542  lvc250f040aaaaaaaaou   lvc250f040aaaaaaaaou
543  lvc250f040afaaaaaaod   lvc250f040afaaaaaaod
544  lvc250f040agaaaaaaod   lvc250f040agaaaaaaod
545  lvc250f040ahaaaaaaod   lvc250f040ahaaaaaaod
546  lvc250f040aiaaaaaaod   lvc250f040aiaaaaaaod
547  lvc250f040ajaaaaaaod   lvc250f040ajaaaaaaod
548  lvc250f040baaaaaaaio   lvc250f040baaaaaaaio
549  lvc250f040baaaaaaaou   lvc250f040baaaaaaaou
550  lvc250f040caaaaaaaio   lvc250f040caaaaaaaio
551  lvc250f040caaaaaaaou   lvc250f040caaaaaaaou
552  lvc250f040daaaaaaaio   lvc250f040daaaaaaaio
553  lvc250f040daaaaaaaou   lvc250f040daaaaaaaou
554  lvc250f040eaaaaaaaio   lvc250f040eaaaaaaaio
555  lvc250f040eaaaaaaaou   lvc250f040eaaaaaaaou
556  lvc250f040faaaaaaaio   lvc250f040faaaaaaaio
557  lvc250f040faaaaaaaou   lvc250f040faaaaaaaou
558  lvc250f040gaaaaaaaio   lvc250f040gaaaaaaaio
559  lvc250f040gaaaaaaaou   lvc250f040gaaaaaaaou
560  lvc250f040haaaaaaaio   lvc250f040haaaaaaaio
561  lvc250f040haaaaaaaou   lvc250f040haaaaaaaou
562  lvc250f080aaaaaaaaio   lvc250f080aaaaaaaaio
563  lvc250f080aaaaaaaaou   lvc250f080aaaaaaaaou
564  lvc250f080afaaaaaaod   lvc250f080afaaaaaaod
565  lvc250f080agaaaaaaod   lvc250f080agaaaaaaod
566  lvc250f080ahaaaaaaod   lvc250f080ahaaaaaaod
567  lvc250f080aiaaaaaaod   lvc250f080aiaaaaaaod
568  lvc250f080ajaaaaaaod   lvc250f080ajaaaaaaod
569  lvc250f080baaaaaaaio   lvc250f080baaaaaaaio
570  lvc250f080baaaaaaaou   lvc250f080baaaaaaaou
571  lvc250f080caaaaaaaio   lvc250f080caaaaaaaio
572  lvc250f080caaaaaaaou   lvc250f080caaaaaaaou
573  lvc250f080daaaaaaaio   lvc250f080daaaaaaaio
574  lvc250f080daaaaaaaou   lvc250f080daaaaaaaou
575  lvc250f080eaaaaaaaio   lvc250f080eaaaaaaaio
576  lvc250f080eaaaaaaaou   lvc250f080eaaaaaaaou
577  lvc250f080faaaaaaaio   lvc250f080faaaaaaaio
578  lvc250f080faaaaaaaou   lvc250f080faaaaaaaou
579  lvc250f080gaaaaaaaio   lvc250f080gaaaaaaaio
580  lvc250f080gaaaaaaaou   lvc250f080gaaaaaaaou
581  lvc250f080haaaaaaaio   lvc250f080haaaaaaaio
582  lvc250f080haaaaaaaou   lvc250f080haaaaaaaou
583  lvc250f120aaaaaaaaio   lvc250f120aaaaaaaaio
584  lvc250f120aaaaaaaaou   lvc250f120aaaaaaaaou
585  lvc250f120afaaaaaaod   lvc250f120afaaaaaaod
586  lvc250f120agaaaaaaod   lvc250f120agaaaaaaod
587  lvc250f120ahaaaaaaod   lvc250f120ahaaaaaaod
588  lvc250f120baaaaaaaio   lvc250f120baaaaaaaio
589  lvc250f120baaaaaaaou   lvc250f120baaaaaaaou
590  lvc250f120caaaaaaaio   lvc250f120caaaaaaaio
591  lvc250f120caaaaaaaou   lvc250f120caaaaaaaou
592  lvc250f120daaaaaaaio   lvc250f120daaaaaaaio
593  lvc250f120daaaaaaaou   lvc250f120daaaaaaaou
594  lvc250f120eaaaaaaaio   lvc250f120eaaaaaaaio
595  lvc250f120eaaaaaaaou   lvc250f120eaaaaaaaou
596  lvc250f120faaaaaaaio   lvc250f120faaaaaaaio
597  lvc250f120faaaaaaaou   lvc250f120faaaaaaaou
598  lvc250f120gaaaaaaaio   lvc250f120gaaaaaaaio
599  lvc250f120gaaaaaaaou   lvc250f120gaaaaaaaou
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[Diff pin]  inv_pin  vdiff  tdelay_typ  tdelay_min  tdelay_max
10   11   0.1   0.0s   0.0s   0.0s
13   14   0.1   0.0s   0.0s   0.0s
16   17   0.1   0.0s   0.0s   0.0s
19   20   0.1   0.0s   0.0s   0.0s
34   35   0.1   0.0s   0.0s   0.0s
38   39   0.1   0.0s   0.0s   0.0s
42   43   0.1   0.0s   0.0s   0.0s
46   47   0.1   0.0s   0.0s   0.0s
84   85   0.1   0.0s   0.0s   0.0s
87   88   0.1   0.0s   0.0s   0.0s
90   91   0.1   0.0s   0.0s   0.0s
93   94   0.1   0.0s   0.0s   0.0s
96   97   0.1   0.0s   0.0s   0.0s
99   100   0.1   0.0s   0.0s   0.0s
102   103   0.1   0.0s   0.0s   0.0s
105   106   0.1   0.0s   0.0s   0.0s
108   109   0.1   0.0s   0.0s   0.0s
111   112   0.1   0.0s   0.0s   0.0s
114   115   0.1   0.0s   0.0s   0.0s
117   118   0.1   0.0s   0.0s   0.0s
120   121   0.1   0.0s   0.0s   0.0s
123   124   0.1   0.0s   0.0s   0.0s
126   127   0.1   0.0s   0.0s   0.0s
129   130   0.1   0.0s   0.0s   0.0s
132   133   0.1   0.0s   0.0s   0.0s
135   136   0.1   0.0s   0.0s   0.0s
138   139   0.1   0.0s   0.0s   0.0s
141   142   0.1   0.0s   0.0s   0.0s
911   912   0.1   0.0s   0.0s   0.0s
913   914   0.1   0.0s   0.0s   0.0s
915   916   0.1   0.0s   0.0s   0.0s
917   918   0.1   0.0s   0.0s   0.0s
919   920   0.1   0.0s   0.0s   0.0s
921   922   0.1   0.0s   0.0s   0.0s
923   924   0.1   0.0s   0.0s   0.0s
925   926   0.1   0.0s   0.0s   0.0s
931   932   0.1   0.0s   0.0s   0.0s
933   934   0.1   0.0s   0.0s   0.0s
935   936   0.1   0.0s   0.0s   0.0s
937   938   0.1   0.0s   0.0s   0.0s
939   940   0.1   0.0s   0.0s   0.0s
941   942   0.1   0.0s   0.0s   0.0s
943   944   0.1   0.0s   0.0s   0.0s
945   946   0.1   0.0s   0.0s   0.0s
954   955   0.1   0.0s   0.0s   0.0s
957   958   0.1   0.0s   0.0s   0.0s
960   961   0.1   0.0s   0.0s   0.0s
963   964   0.1   0.0s   0.0s   0.0s
966   967   0.1   0.0s   0.0s   0.0s
969   970   0.1   0.0s   0.0s   0.0s
972   973   0.1   0.0s   0.0s   0.0s
975   976   0.1   0.0s   0.0s   0.0s
978   979   0.1   0.0s   0.0s   0.0s
981   982   0.1   0.0s   0.0s   0.0s
984   985   0.1   0.0s   0.0s   0.0s
987   988   0.1   0.0s   0.0s   0.0s
994   995   0.1   0.0s   0.0s   0.0s
997   998   0.1   0.0s   0.0s   0.0s
1000   1001   0.1   0.0s   0.0s   0.0s
1003   1004   0.1   0.0s   0.0s   0.0s
1006   1007   0.1   0.0s   0.0s   0.0s
1009   1010   0.1   0.0s   0.0s   0.0s
1012   1013   0.1   0.0s   0.0s   0.0s
1015   1016   0.1   0.0s   0.0s   0.0s
1018   1019   0.1   0.0s   0.0s   0.0s
1021   1022   0.1   0.0s   0.0s   0.0s
1024   1025   0.1   0.0s   0.0s   0.0s
1027   1028   0.1   0.0s   0.0s   0.0s
1030   1031   0.1   0.0s   0.0s   0.0s
1033   1034   0.1   0.0s   0.0s   0.0s
1036   1037   0.1   0.0s   0.0s   0.0s
1039   1040   0.1   0.0s   0.0s   0.0s
1044   1045   0.1   0.0s   0.0s   0.0s
1047   1048   0.1   0.0s   0.0s   0.0s
1050   1051   0.1   0.0s   0.0s   0.0s
1053   1054   0.1   0.0s   0.0s   0.0s
1056   1057   0.1   0.0s   0.0s   0.0s
1059   1060   0.1   0.0s   0.0s   0.0s
1062   1063   0.1   0.0s   0.0s   0.0s
1065   1066   0.1   0.0s   0.0s   0.0s
1068   1069   0.1   0.0s   0.0s   0.0s
1071   1072   0.1   0.0s   0.0s   0.0s
1074   1075   0.1   0.0s   0.0s   0.0s
1077   1078   0.1   0.0s   0.0s   0.0s
1080   1081   0.1   0.0s   0.0s   0.0s
1083   1084   0.1   0.0s   0.0s   0.0s
1086   1087   0.1   0.0s   0.0s   0.0s
1089   1090   0.1   0.0s   0.0s   0.0s
1092   1093   0.1   0.0s   0.0s   0.0s
1095   1096   0.1   0.0s   0.0s   0.0s
1098   1099   0.1   0.0s   0.0s   0.0s
1101   1102   0.1   0.0s   0.0s   0.0s
1149   1150   0.1   0.0s   0.0s   0.0s
1151   1152   0.1   0.0s   0.0s   0.0s
1153   1154   0.1   0.0s   0.0s   0.0s
1155   1156   0.1   0.0s   0.0s   0.0s
1161   1162   0.1   0.0s   0.0s   0.0s
1163   1164   0.1   0.0s   0.0s   0.0s
1165   1166   0.1   0.0s   0.0s   0.0s
1167   1168   0.1   0.0s   0.0s   0.0s
1388   1389   0.1   0.0s   0.0s   0.0s
1391   1392   0.1   0.0s   0.0s   0.0s
1394   1395   0.1   0.0s   0.0s   0.0s
1397   1398   0.1   0.0s   0.0s   0.0s
1447   1448   0.1   0.0s   0.0s   0.0s
1449   1450   0.1   0.0s   0.0s   0.0s
1451   1452   0.1   0.0s   0.0s   0.0s
1453   1454   0.1   0.0s   0.0s   0.0s
1468   1469   0.1   0.0s   0.0s   0.0s
1472   1473   0.1   0.0s   0.0s   0.0s
1476   1477   0.1   0.0s   0.0s   0.0s
1480   1481   0.1   0.0s   0.0s   0.0s
1492   1493   0.1   0.0s   0.0s   0.0s
1496   1497   0.1   0.0s   0.0s   0.0s
1500   1501   0.1   0.0s   0.0s   0.0s
1504   1505   0.1   0.0s   0.0s   0.0s
| Models and submodels in the file (1471): blv250axxxafaaaaaain (Input), blv250axxxafaaaabain (Input), blv250axxxagaaaaaain (Input), blv250axxxagaaaabain (Input), blv250axxxefaaaaaain (Input), blv250axxxefaaaabain (Input), blv250axxxegaaaaaain (Input), blv250axxxegaaaabain (Input), blv250f160aaaaaaaaio (I/O), blv250f160aaaaaaaaou (Output), blv250f160eaaaaaaaio (I/O), blv250f160eaaaaaaaou (Output), blv250s160aaaaaaaaio (I/O), blv250s160aaaaaaaaou (Output), blv250s160eaaaaaaaio (I/O), blv250s160eaaaaaaaou (Output), h1d180axxxafaaaaaain (Input), h1d180axxxafaaaabain (Input), h1d180axxxagaaaaaain (Input), h1d180axxxagaaaabain (Input), h1d180axxxahaaaaaain (Input), h1d180axxxahaaaabain (Input), h1d180axxxefaaaaaain (Input), h1d180axxxefaaaabain (Input), h1d180axxxegaaaaaain (Input), h1d180axxxegaaaabain (Input), h1d180axxxehaaaaaain (Input), h1d180axxxehaaaabain (Input), h1d180f080aaaaaaaaio (I/O), h1d180f080aaaaaaaaou (Output), h1d180f080aaaaaabaio (I/O), h1d180f080eaaaaaaaio (I/O), h1d180f080eaaaaaaaou (Output), h1d180f080eaaaaabaio (I/O), h1d180s080aaaaaaaaio (I/O), h1d180s080aaaaaaaaou (Output), h1d180s080aaaaaabaio (I/O), h1d180s080eaaaaaaaio (I/O), h1d180s080eaaaaaaaou (Output), h1d180s080eaaaaabaio (I/O), h2d180axxxafaaaaaain (Input), h2d180axxxafaaaabain (Input), h2d180axxxagaaaaaain (Input), h2d180axxxagaaaabain (Input), h2d180axxxahaaaaaain (Input), h2d180axxxahaaaabain (Input), h2d180axxxefaaaaaain (Input), h2d180axxxefaaaabain (Input), h2d180axxxegaaaaaain (Input), h2d180axxxegaaaabain (Input), h2d180axxxehaaaaaain (Input), h2d180axxxehaaaabain (Input), hs1180axxxafaaaaaain (Input), hs1180axxxagaaaaaain (Input), hs1180axxxahaaaaaain (Input), hs1180axxxefaaaaaain (Input), hs1180axxxegaaaaaain (Input), hs1180axxxehaaaaaain (Input), hs1180f080aaaaaaaaio (I/O), hs1180f080aaaaaaaaou (Output), hs1180f080eaaaaaaaio (I/O), hs1180f080eaaaaaaaou (Output), hs1180s080aaaaaaaaio (I/O), hs1180s080aaaaaaaaou (Output), hs1180s080eaaaaaaaio (I/O), hs1180s080eaaaaaaaou (Output), hs2180axxxafaaaaaain (Input), hs2180axxxagaaaaaain (Input), hs2180axxxahaaaaaain (Input), hs2180axxxefaaaaaain (Input), hs2180axxxegaaaaaain (Input), hs2180axxxehaaaaaain (Input), ltd330axxxafaaaaaain (Input), ltd330axxxefaaaaaain (Input), ltd330f040aaaaaaaaio (I/O), ltd330f040aaaaaaaaou (Output), ltd330f040eaaaaaaaio (I/O), ltd330f040eaaaaaaaou (Output), ltd330f080aaaaaaaaio (I/O), ltd330f080aaaaaaaaou (Output)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
